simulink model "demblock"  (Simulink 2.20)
settings: Solver=FixedStepDiscrete  StartTime=0.0  StopTime=tmax  MaxStep=tmax/200  RelTol=1e-3  AbsTol=1e-3

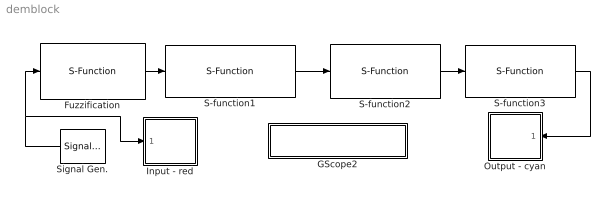
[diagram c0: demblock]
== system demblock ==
  Fuzzification : S-Function  FunctionName=sfunfuzz  Parameters=figno,mfs,rdom,idom  PortCounts=[]  SFunctionModules=''  mask(Fuzzification){}
      mask help: Fuzzification
      mask init:
      | figno = @1; mfs = @2; rdom = @3; idom = @4;
  GScope2 : Subsystem  mask(Pause){}
      mask help: Pause
      mask init:
      | sec  = @1;
  Input - red : Subsystem  mask(Graph scope.){}
      mask help: Graph scope using MATLAB graph window. Enter figure, plotting ranges and line type.
      mask init:
      | figno = @1; color = @5; ax = [0, @2, @3, @4];
  Output - cyan : Subsystem  Orientation=left  mask(Graph scope.){}
      mask help: Graph scope using MATLAB graph window. Enter figure, plotting ranges and line type.
      mask init:
      | figno = @1; color = @5; ax = [0, @2, @3, @4];
  S-function1 : S-Function  FunctionName=sfunimpl  Parameters=figno, fs, domain, impl, par  PortCounts=[]  SFunctionModules=''  mask(Implication){}
      mask help: Implication
      mask init:
      | figno = @1; fs = @2; domain = @3; impl = @4; par = @5;
  S-function2 : S-Function  FunctionName=sfunagr  Parameters=figno, nsets, domain, agr, par  PortCounts=[]  SFunctionModules=''  mask(Agregation){}
      mask help: Aggregation
      mask init:
      | figno = @1; nsets = @2; domain = @3; agr = @4; par = @5;
  S-function3 : S-Function  FunctionName=sfundef  Parameters=figno,domain, def, par1, par2  PortCounts=[]  SFunctionModules=''  mask(Defuzzification){}
      mask help: Dufuzzification
      mask init:
      | figno = @1; domain = @2; def = @3; par1 = @4; par2 = @5;
  Signal Gen. : SignalGenerator  Orientation=left  WaveForm=sine  Amplitude=1.000000  Frequency=3.000000  Units=rad/sec
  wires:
  S-function1/1 -> S-function2/1
  S-function2/1 -> S-function3/1
  S-function3/1 -> Output - cyan/1(x)
  Fuzzification/1 -> S-function1/1
  Signal Gen./1 -> Fuzzification/1, Input - red/1(x)

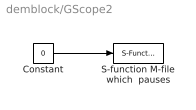
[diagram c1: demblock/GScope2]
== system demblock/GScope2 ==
  Constant : Constant  Value=0
  S-function M-file which  pauses : S-Function  FunctionName=sfunpaus  Parameters=sec  PortCounts=[]  SFunctionModules=''
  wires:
  Constant/1 -> S-function M-file which  pauses/1

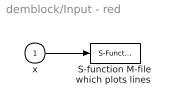
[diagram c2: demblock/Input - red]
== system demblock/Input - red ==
  x : Inport  Port=1  PortWidth=-1  SampleTime=-1
  "S-function M-file which plots lines " : S-Function  FunctionName=sfunplot  Parameters=figno,ax, color  PortCounts=[]  SFunctionModules=''
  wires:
  x/1 -> "S-function M-file which plots lines "/1

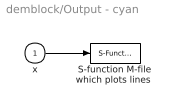
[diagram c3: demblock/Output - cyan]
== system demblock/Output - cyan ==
  x : Inport  Port=1  PortWidth=-1  SampleTime=-1
  "S-function M-file which plots lines " : S-Function  FunctionName=sfunplot  Parameters=figno,ax, color  PortCounts=[]  SFunctionModules=''
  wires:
  x/1 -> "S-function M-file which plots lines "/1
